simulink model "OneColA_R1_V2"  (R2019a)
settings: Solver=ode15s  StartTime=0.0  StopTime=tend  RelTol=1e-3
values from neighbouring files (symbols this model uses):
  Extract_J = zeros(83,1)'    [Simulate1Col.m]    (also in Simulate1Col_OL.m; Simulate1Col_R1.m; Simulate1Col_R2.m)
  Extract_xB = zeros(82,1)'    [Simulate1Col.m]    (also in Simulate1Col_OL.m; Simulate1Col_R1.m; Simulate1Col_R2.m)
  Extract_xD = zeros(82,1)'    [Simulate1Col.m]    (also in Simulate1Col_OL.m; Simulate1Col_R1.m; Simulate1Col_R2.m)
  F0 = 1    [colamod.m]    (also in ColumnA_simulation.m; Simulate1Col.m = F; Simulate1Col_OL.m = F; Simulate1Col_R1.m = F)
  F0step = 0.05    [Simulate1Col.m]    (also in Simulate1Col_OL.m = 1*F0*.1; Simulate1Col_R1.m; Simulate1Col_R2.m = 0.15)
  F0step2 = 0*(0.15-F0step)    (= 0)    [Simulate1Col.m]    (also in Simulate1Col_R1.m; Simulate1Col_R2.m = 0.1)
  F0step2_t = 30    [Simulate1Col.m]    (also in Simulate1Col_R1.m; Simulate1Col_R2.m = 80)
  F0step_t = 10    [Simulate1Col.m]    (also in Simulate1Col_OL.m; Simulate1Col_R1.m; Simulate1Col_R2.m)
  LT0 = u_opt(1)    [Simulate1Col.m]    (also in Simulate1Col_OL.m; Simulate1Col_R1.m; Simulate1Col_R2.m)
  pV0 = pV    [Simulate1Col.m]    (also in Simulate1Col_OL.m; Simulate1Col_R1.m; Simulate1Col_R2.m)
  pVstep = 0.02    [Simulate1Col.m]    (also in Simulate1Col_OL.m = 0*(0.13-pV0); Simulate1Col_R1.m; Simulate1Col_R2.m = 0.06)
  pVstept = 50    [Simulate1Col.m]    (also in Simulate1Col_OL.m; Simulate1Col_R1.m; Simulate1Col_R2.m)
  qF = U(7)    [colamod.m]    (also in ColumnA_simulation.m; Simulate1Col.m = 1; Simulate1Col_OL.m = 1; Simulate1Col_R1.m = 1)
  VB0 = u_opt(2)    [Simulate1Col.m]    (also in Simulate1Col_OL.m; Simulate1Col_R1.m; Simulate1Col_R2.m)
  x0 = 0.5*ones(1,82)'    [col_obj.m]    (also in Simulate1Col.m = x; Simulate1Col_OL.m = x; Simulate1Col_R1.m = x; Simulate1Col_R2.m = x)
  xBsp = 0.95    [Simulate1Col.m]    (also in Simulate1Col_OL.m; Simulate1Col_R1.m; Simulate1Col_R2.m)
  xDmin = 0.95    [Simulate1Col.m]    (also in Simulate1Col_OL.m; Simulate1Col_R1.m; Simulate1Col_R2.m)
  zF = U(6)    [colamod.m]    (also in ColumnA_simulation.m; Simulate1Col.m = 0.5; Simulate1Col_OL.m = 0.5; Simulate1Col_R1.m = 0.5)
undefined symbols (not defined in the file or in its folder): Calc_xDsp, ColumnA_simulation, extract, KxB, KxD, tauIxB, tauIxD, TxB, TxD
libraries: simulink x1

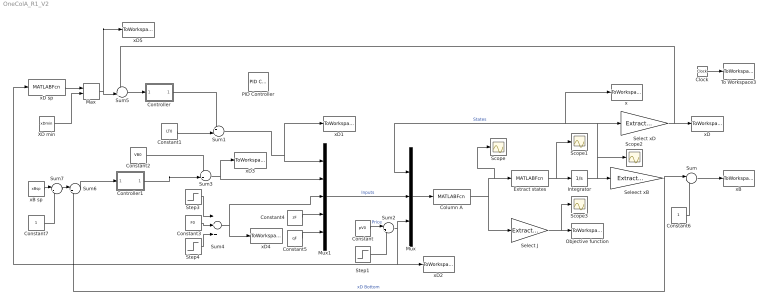
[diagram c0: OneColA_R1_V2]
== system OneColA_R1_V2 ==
  Clock : Clock
  Column A : MATLABFcn  MATLABFcn=ColumnA_simulation(u)  OutputDimensions=83
  Constant : Constant  Value=pV0
  Constant1 : Constant  Value=LT0
  Constant2 : Constant  Value=VB0
  Constant3 : Constant  Value=F0
  Constant4 : Constant  Value=zF
  Constant5 : Constant  Value=qF
  Constant6 : Constant
  Constant7 : Constant
  Controller : Subsystem
  Controller1 : Subsystem
  Extract states : MATLABFcn  MATLABFcn=extract(u)  OutputDimensions=82
  Integrator : Integrator  InitialCondition=x0
  Max : MinMax  Function=max  Inputs=2
  Mux : Mux  Inputs=3
  Mux1 : Mux  Inputs=5
  Objective function : ToWorkspace  VariableName=Jactual  SampleTime=-1
  PID Controller : simulink/Continuous/PID Controller  Controller=PID  Form=Parallel  TimeDomain=Continuous-time  SampleTime=-1  IntegratorMethod=Forward Euler  FilterMethod=Forward Euler  ControllerParametersSource=internal  P=1  I=1  D=0  UseFilter=on  N=100  TunerSelectOption=Transfer Function Based (PID Tuner App)  InitialConditionSource=internal  InitialConditionForIntegrator=0  InitialConditionForFilter=0  DifferentiatorICPrevScaledInput=0  ExternalReset=none  TrackingMode=off  Kt=1  LimitOutput=off  UpperSaturationLimit=inf  LowerSaturationLimit=-inf  LinearizeAsGain=on  AntiWindupMode=none  Kb=1  POutMin=[]  POutMax=[]  IOutMin=[]  IOutMax=[]  DOutMin=[]  DOutMax=[]  NOutMin=[]  NOutMax=[]  SumOutMin=[]  SumOutMax=[]  SaturationOutMin=[]  SaturationOutMax=[]  PParamMin=[]  PParamMax=[]  IParamMin=[]  IParamMax=[]  DParamMin=[]  DParamMax=[]  NParamMin=[]  NParamMax=[]  KbParamMin=[]  KbParamMax=[]  KtParamMin=[]  KtParamMax=[]  KbOutMin=[]  KbOutMax=[]  KtOutMin=[]  KtOutMax=[]  IntegratorOutMin=[]  IntegratorOutMax=[]  FilterOutMin=[]  FilterOutMax=[]  SumI1OutMin=[]  SumI1OutMax=[]  SumI2OutMin=[]  SumI2OutMax=[]  SumI3OutMin=[]  SumI3OutMax=[]  SumI4OutMin=[]  SumI4OutMax=[]  SumDOutMin=[]  SumDOutMax=[]  DifferentiatorOutMin=[]  DifferentiatorOutMax=[]  FilterDiffOutCoefMin=[]  FilterDiffOutCoefMax=[]  ReciprocalOutMin=[]  ReciprocalOutMax=[]  SumDenOutMin=[]  SumDenOutMax=[]  SumNumOutMin=[]  SumNumOutMax=[]  DivideOutMin=[]  DivideOutMax=[]  IntegratorContinuousStateAttributes=''  IntegratorStateMustResolveToSignalObject=off  IntegratorRTWStateStorageClass=Auto  FilterContinuousStateAttributes=''  FilterStateMustResolveToSignalObject=off  FilterRTWStateStorageClass=Auto  ParallelPVariant=InternalParameters  IdealPVariant=Disabled  IVariant=InternalParameters  DVariant=InternalParameters  IntegratorVariant=Continuous  SatVariant=Disabled  AWVariant=Passthrough  PCopyVariant=Disabled  TRVariant=Disabled  FdbkBlocksVariant=Forward  IdealPFdbkVariant=Disabled  SatFdbkVariant=Disabled  DerivativeFilterVariant=ContFilter  NVariant=InternalParameters  NCopyVariant=Disabled  FilterICVariant=InternalICsFilter  IntegratorICVariant=InternalICs  ExternalResetVariant=Disabled  TRSumVariant=Passthrough  SumFdbkVariant=Disabled  SumVariant=Sum_PID
  Scope{,1..3} (4 alike) : Scope
  Select J : Gain  Gain=Extract_J  Multiplication=Matrix(K*u)
  Select xD : Gain  Gain=Extract_xD  Multiplication=Matrix(K*u)
  Seleect xB : Gain  Gain=Extract_xB  Multiplication=Matrix(K*u)
  Step1 : Step  Time=pVstept  After=pVstep  SampleTime=0
  Step3 : Step  Time=F0step_t  After=F0step  SampleTime=0
  Step4 : Step  Time=F0step2_t  After=F0step2  SampleTime=0
  Sum : Sum  Inputs=|-+
  Sum1 : Sum  Inputs=++|
  Sum2 : Sum  Inputs=|++
  Sum3 : Sum  Inputs=++|
  Sum4 : Sum  Inputs=+++
  Sum5 : Sum  Inputs=-+|
  Sum6 : Sum  Inputs=|+-
  Sum7 : Sum  Inputs=|-+
  To Workspace3 : ToWorkspace  VariableName=time  SampleTime=-1
  XD min : Constant  Value=xDmin
  x : ToWorkspace  VariableName=States  SampleTime=-1
  xB : ToWorkspace  VariableName=xB  SampleTime=-1
  xB sp : Constant  Value=xBsp
  xD : ToWorkspace  VariableName=xD  SampleTime=-1
  xD sp : MATLABFcn  MATLABFcn=Calc_xDsp(u)  OutputDimensions=1
  xD1 : ToWorkspace  VariableName=LT  SampleTime=-1
  xD2 : ToWorkspace  VariableName=pV  SampleTime=-1
  xD3 : ToWorkspace  VariableName=VB  SampleTime=-1
  xD4 : ToWorkspace  VariableName=Fin  SampleTime=-1
  xD5 : ToWorkspace  VariableName=xDsp  SampleTime=-1
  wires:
  Mux/1 -> Column A/1
  Mux1/1 -> Mux/2  "Inputs"
  Constant4/1 -> Mux1/4
  Constant5/1 -> Mux1/5
  Column A/1 -> Select J/1, Extract states/1, Scope/1
  Extract states/1 -> Scope1/1, Integrator/1
  Integrator/1 -> Seleect xB/1, Select xD/1, x/1, Mux/1, Scope2/1  "States"
  Select xD/1 -> Sum5/1, xD/1
  Select J/1 -> Scope3/1, Objective function/1
  Clock/1 -> To Workspace3/1
  Seleect xB/1 -> Sum/1, Sum6/2  "xD Bottom"
  Sum/1 -> xB/1
  Constant6/1 -> Sum/2
  Sum1/1 -> xD1/1, Mux1/1
  Sum2/1 -> xD2/1, xD sp/1, Mux/3
  Constant/1 -> Sum2/1  "Price"
  Sum3/1 -> Mux1/2, xD3/1
  Constant3/1 -> Sum4/2
  Sum4/1 -> xD4/1, Mux1/3
  Step3/1 -> Sum4/1
  Step1/1 -> Sum2/2
  Step4/1 -> Sum4/3
  Constant2/1 -> Sum3/1
  Constant1/1 -> Sum1/2
  Controller1/1(u) -> Sum3/2
  Sum6/1 -> Controller1/1(error)
  Max/1 -> xD5/1, Sum5/2
  xD sp/1 -> Max/1
  XD min/1 -> Max/2
  Sum5/1 -> Controller/1(error)
  Controller/1(u) -> Sum1/1
  xB sp/1 -> Sum7/1
  Sum7/1 -> Sum6/1
  Constant7/1 -> Sum7/2

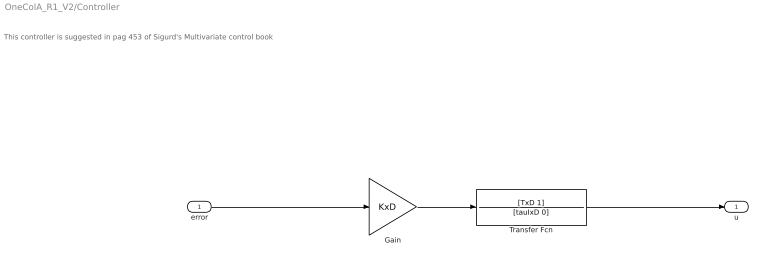
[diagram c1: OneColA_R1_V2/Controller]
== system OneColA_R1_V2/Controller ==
  note: This controller is suggested in pag 453 of Sigurd's Multivariate control book
  error : Inport
  Gain : Gain  Gain=KxD
  Transfer Fcn : TransferFcn  Numerator=[TxD 1]  Denominator=[tauIxD 0]
  u : Outport
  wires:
  Gain/1 -> Transfer Fcn/1
  error/1 -> Gain/1
  Transfer Fcn/1 -> u/1

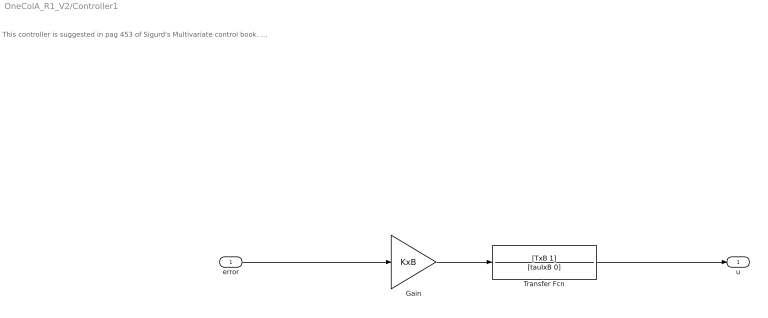
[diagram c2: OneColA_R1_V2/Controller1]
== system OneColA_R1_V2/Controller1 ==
  note: This controller is suggested in pag 453 of Sigurd's Multivariate control book. Here we are controlling xB=0.95. In the book, and the original model, xB is related to the concentration of the light component in the bottom (that is why it is 1-xB^sp
  error : Inport
  Gain : Gain  Gain=KxB
  Transfer Fcn : TransferFcn  Numerator=[TxB 1]  Denominator=[tauIxB 0]
  u : Outport
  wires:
  Gain/1 -> Transfer Fcn/1
  error/1 -> Gain/1
  Transfer Fcn/1 -> u/1
